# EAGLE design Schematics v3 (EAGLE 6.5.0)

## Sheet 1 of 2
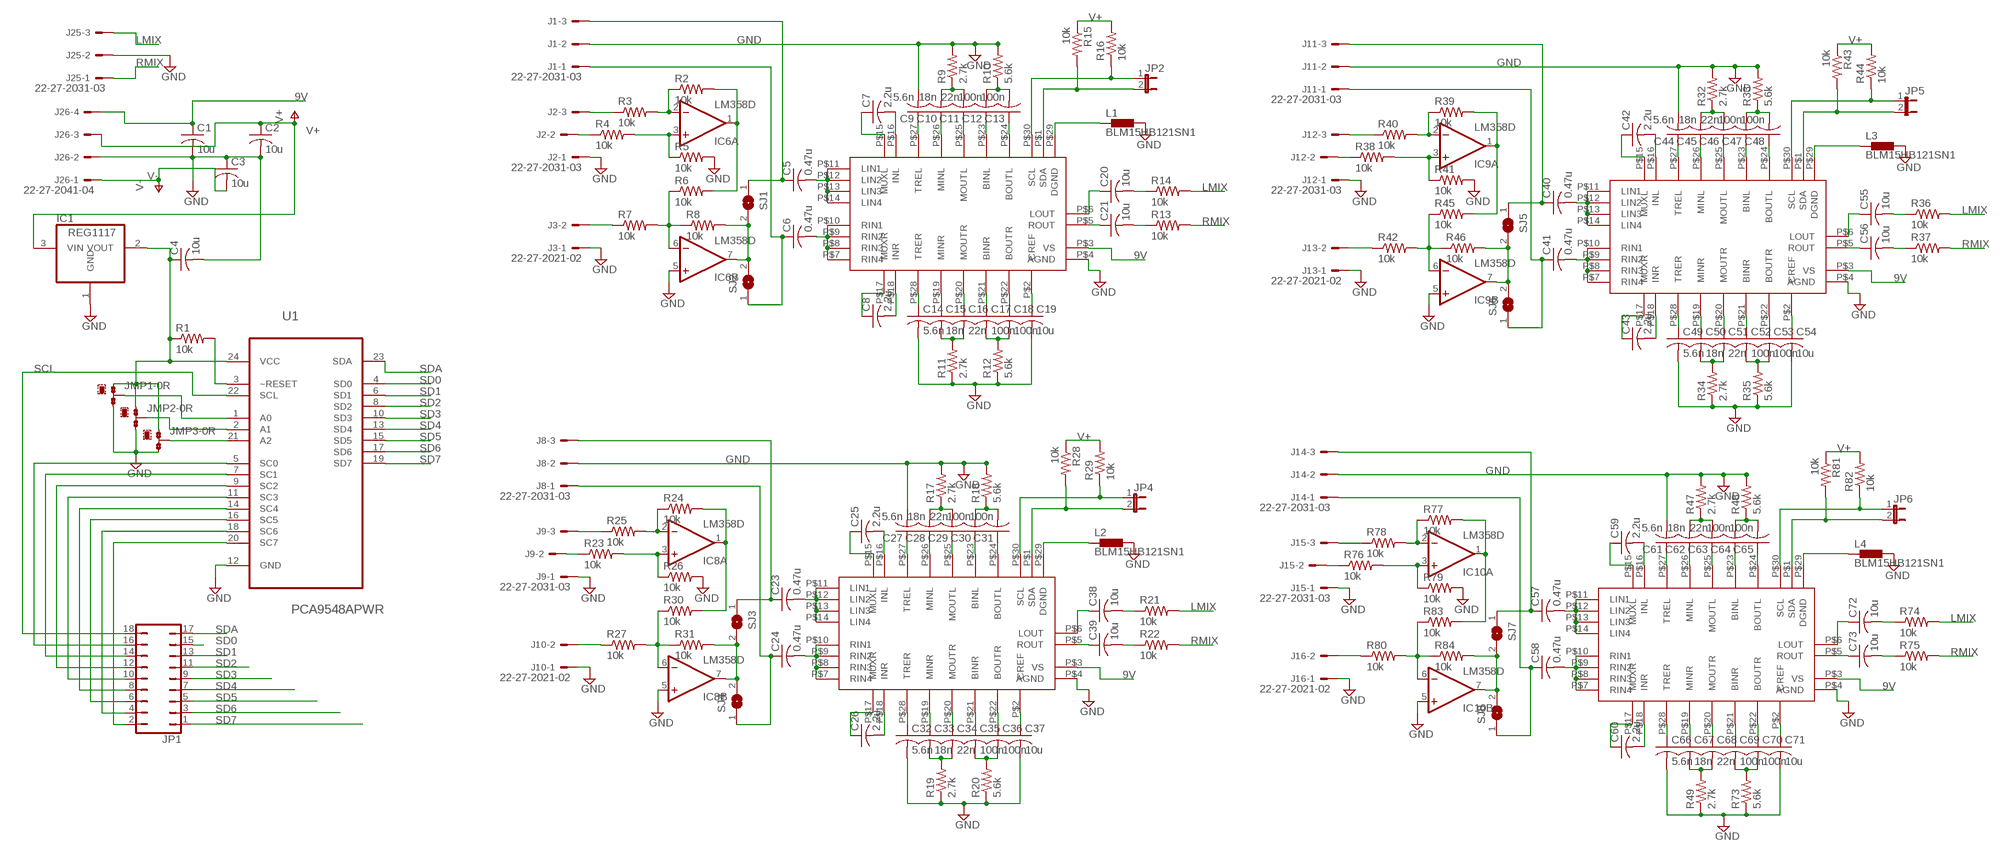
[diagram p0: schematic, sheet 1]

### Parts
C1  10u  C-USC1206  [C1206]
C2  10u  C-USC1206  [C1206]
C3  10u  C-USC1206  [C1206]
C4  10u  C-USC1206  [C1206]
C5  0.47u  C-USC1206  [C1206]
C6  0.47u  C-USC1206  [C1206]
C7  2.2u  C-USC1206  [C1206]
C8  2.2u  C-USC1206  [C1206]
C9  5.6n  C-USC1206  [C1206]
C10  18n  C-USC1206  [C1206]
C11  22n  C-USC1206  [C1206]
C12  100n  C-USC1206  [C1206]
C13  100n  C-USC1206  [C1206]
C14  5.6n  C-USC1206  [C1206]
C15  18n  C-USC1206  [C1206]
C16  22n  C-USC1206  [C1206]
C17  100n  C-USC1206  [C1206]
C18  100n  C-USC1206  [C1206]
C19  10u  C-USC1206  [C1206]
C20  10u  C-USC1206  [C1206]
C21  10u  C-USC1206  [C1206]
C23  0.47u  C-USC1206  [C1206]
C24  0.47u  C-USC1206  [C1206]
C25  2.2u  C-USC1206  [C1206]
C26  2.2u  C-USC1206  [C1206]
C27  5.6n  C-USC1206  [C1206]
C28  18n  C-USC1206  [C1206]
C29  22n  C-USC1206  [C1206]
C30  100n  C-USC1206  [C1206]
C31  100n  C-USC1206  [C1206]
C32  5.6n  C-USC1206  [C1206]
C33  18n  C-USC1206  [C1206]
C34  22n  C-USC1206  [C1206]
C35  100n  C-USC1206  [C1206]
C36  100n  C-USC1206  [C1206]
C37  10u  C-USC1206  [C1206]
C38  10u  C-USC1206  [C1206]
C39  10u  C-USC1206  [C1206]
C40  0.47u  C-USC1206  [C1206]
C41  0.47u  C-USC1206  [C1206]
C42  2.2u  C-USC1206  [C1206]
C43  2.2u  C-USC1206  [C1206]
C44  5.6n  C-USC1206  [C1206]
C45  18n  C-USC1206  [C1206]
C46  22n  C-USC1206  [C1206]
C47  100n  C-USC1206  [C1206]
C48  100n  C-USC1206  [C1206]
C49  5.6n  C-USC1206  [C1206]
C50  18n  C-USC1206  [C1206]
C51  22n  C-USC1206  [C1206]
C52  100n  C-USC1206  [C1206]
C53  100n  C-USC1206  [C1206]
C54  10u  C-USC1206  [C1206]
C55  10u  C-USC1206  [C1206]
C56  10u  C-USC1206  [C1206]
C57  0.47u  C-USC1206  [C1206]
C58  0.47u  C-USC1206  [C1206]
C59  2.2u  C-USC1206  [C1206]
C60  2.2u  C-USC1206  [C1206]
C61  5.6n  C-USC1206  [C1206]
C62  18n  C-USC1206  [C1206]
C63  22n  C-USC1206  [C1206]
C64  100n  C-USC1206  [C1206]
C65  100n  C-USC1206  [C1206]
C66  5.6n  C-USC1206  [C1206]
C67  18n  C-USC1206  [C1206]
C68  22n  C-USC1206  [C1206]
C69  100n  C-USC1206  [C1206]
C70  100n  C-USC1206  [C1206]
C71  10u  C-USC1206  [C1206]
C72  10u  C-USC1206  [C1206]
C73  10u  C-USC1206  [C1206]
IC1  REG1117  [SOT223]
IC6  LM358D  [SO08]
IC8  LM358D  [SO08]
IC9  LM358D  [SO08]
IC10  LM358D  [SO08]
J1  22-27-2031-03  [6410-03]
J2  22-27-2031-03  [6410-03]
J3  22-27-2021-02  [6410-02]
J8  22-27-2031-03  [6410-03]
J9  22-27-2031-03  [6410-03]
J10  22-27-2021-02  [6410-02]
J11  22-27-2031-03  [6410-03]
J12  22-27-2031-03  [6410-03]
J13  22-27-2021-02  [6410-02]
J14  22-27-2031-03  [6410-03]
J15  22-27-2031-03  [6410-03]
J16  22-27-2021-02  [6410-02]
J25  22-27-2031-03  [6410-03]
J26  22-27-2041-04  [6410-04]
JMP1  0R-JUMPB  [B0R-JMP]
JMP2  0R-JUMPB  [B0R-JMP]
JMP3  0R-JUMPB  [B0R-JMP]
JP1  JP9Q  [JP9Q]
JP2  JP1E  [JP1]
JP4  JP1E  [JP1]
JP5  JP1E  [JP1]
JP6  JP1E  [JP1]
L1  BLM15HB121SN1  [0402]
L2  BLM15HB121SN1  [0402]
L3  BLM15HB121SN1  [0402]
L4  BLM15HB121SN1  [0402]
R1  10k  R-US_R1206  [R1206]
R2  10k  R-US_R1206  [R1206]
R3  10k  R-US_R1206  [R1206]
R4  10k  R-US_R1206  [R1206]
R5  10k  R-US_R1206  [R1206]
R6  10k  R-US_R1206  [R1206]
R7  10k  R-US_R1206  [R1206]
R8  10k  R-US_R1206  [R1206]
R9  2.7k  R-US_R1206  [R1206]
R10  5.6k  R-US_R1206  [R1206]
R11  2.7k  R-US_R1206  [R1206]
R12  5.6k  R-US_R1206  [R1206]
R13  10k  R-US_R1206  [R1206]
R14  10k  R-US_R1206  [R1206]
R15  10k  R-US_R1206  [R1206]
R16  10k  R-US_R1206  [R1206]
R17  2.7k  R-US_R1206  [R1206]
R18  5.6k  R-US_R1206  [R1206]
R19  2.7k  R-US_R1206  [R1206]
R20  5.6k  R-US_R1206  [R1206]
R21  10k  R-US_R1206  [R1206]
R22  10k  R-US_R1206  [R1206]
R23  10k  R-US_R1206  [R1206]
R24  10k  R-US_R1206  [R1206]
R25  10k  R-US_R1206  [R1206]
R26  10k  R-US_R1206  [R1206]
R27  10k  R-US_R1206  [R1206]
R28  10k  R-US_R1206  [R1206]
R29  10k  R-US_R1206  [R1206]
R30  10k  R-US_R1206  [R1206]
R31  10k  R-US_R1206  [R1206]
R32  2.7k  R-US_R1206  [R1206]
R33  5.6k  R-US_R1206  [R1206]
R34  2.7k  R-US_R1206  [R1206]
R35  5.6k  R-US_R1206  [R1206]
R36  10k  R-US_R1206  [R1206]
R37  10k  R-US_R1206  [R1206]
R38  10k  R-US_R1206  [R1206]
R39  10k  R-US_R1206  [R1206]
R40  10k  R-US_R1206  [R1206]
R41  10k  R-US_R1206  [R1206]
R42  10k  R-US_R1206  [R1206]
R43  10k  R-US_R1206  [R1206]
R44  10k  R-US_R1206  [R1206]
R45  10k  R-US_R1206  [R1206]
R46  10k  R-US_R1206  [R1206]
R47  2.7k  R-US_R1206  [R1206]
R48  5.6k  R-US_R1206  [R1206]
R49  2.7k  R-US_R1206  [R1206]
R73  5.6k  R-US_R1206  [R1206]
R74  10k  R-US_R1206  [R1206]
R75  10k  R-US_R1206  [R1206]
R76  10k  R-US_R1206  [R1206]
R77  10k  R-US_R1206  [R1206]
R78  10k  R-US_R1206  [R1206]
R79  10k  R-US_R1206  [R1206]
R80  10k  R-US_R1206  [R1206]
R81  10k  R-US_R1206  [R1206]
R82  10k  R-US_R1206  [R1206]
R83  10k  R-US_R1206  [R1206]
R84  10k  R-US_R1206  [R1206]
SJ1  SJ  [SJ]
SJ2  SJ  [SJ]
SJ3  SJ  [SJ]
SJ4  SJ  [SJ]
SJ5  SJ  [SJ]
SJ6  SJ  [SJ]
SJ7  SJ  [SJ]
SJ8  SJ  [SJ]
U1  PCA9548APWR  [SOP65P640X120-24N]
U$1  TDA7439  [SDIP30]
U$2  TDA7439  [SDIP30]
U$3  TDA7439  [SDIP30]
U$4  TDA7439  [SDIP30]

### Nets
3.3V: C4.1 IC1.2(VOUT) JMP1.1 JMP2.1 JMP3.1 R1.1 U1.24(VCC)
9V: C1.1 J26.4 U$1.P$3(VS) U$2.P$3(VS) U$3.P$3(VS) U$4.P$3(VS) ; also sheet 2
A0: JMP1.2 U1.1(A0)
A1: JMP2.2 U1.2(A1)
A2: JMP3.2 U1.21(A2)
GND: C1.2 C2.2 C3.1 C4.2 C9.2 C14.2 C19.2 C27.2 C32.2 C37.2 C44.2 C49.2 C54.2 C61.2 C66.2 C71.2 IC1.1(GND) IC6.5(B:+IN) IC8.5(B:+IN) IC9.5(B:+IN) IC10.5(B:+IN) J1.2 J2.1 J3.1 J8.2 J9.1 J10.1 J11.2 J12.1 J13.1 J14.2 J15.1 J16.1 J25.2 J26.2 JMP1.3 JMP2.3 JMP3.3 L1.2 L2.2 L3.2 L4.2 R5.2 R9.2 R10.2 R11.1 R12.1 R17.2 R18.2 R19.1 R20.1 R26.2 R32.2 R33.2 R34.1 R35.1 R41.2 R47.2 R48.2 R49.1 R73.1 R79.2 U1.12(GND) U$1.P$4(AGND) U$2.P$4(AGND) U$3.P$4(AGND) U$4.P$4(AGND) ; also sheet 2
LMIX: J25.3 R14.2 R21.2 R36.2 R74.2 ; also sheet 2
N$1: J2.2 R4.1
N$2: J2.3 R3.1
N$3: IC6.2(A:-IN) R2.1 R3.2
N$4: IC6.3(A:+IN) R4.2 R5.1
N$5: IC6.1(A:OUT) R2.2 R6.2
N$6: IC6.6(B:-IN) R6.1 R7.2 R8.1
N$7: J3.2 R7.1
N$8: IC6.7(B:OUT) R8.2 SJ1.2 SJ2.2
N$9: C5.1 J1.3 SJ1.1
N$10: C6.1 J1.1 SJ2.1
N$11: C5.2 U$1.P$11(LIN1) U$1.P$12(LIN2) U$1.P$13(LIN3) U$1.P$14(LIN4)
N$12: C6.2 U$1.P$7(RIN4) U$1.P$8(RIN3) U$1.P$9(RIN2) U$1.P$10(RIN1)
N$13: C7.1 U$1.P$15(MUXL)
N$14: C7.2 U$1.P$16(INL)
N$15: C9.1 U$1.P$27(TREL)
N$16: C10.1 U$1.P$26(MINL)
N$17: C11.1 U$1.P$25(MOUTL)
N$18: C12.1 U$1.P$23(BINL)
N$19: C13.1 U$1.P$24(BOUTL)
N$20: C10.2 C11.2 R9.1
N$21: C12.2 C13.2 R10.1
N$22: C8.1 U$1.P$17(MUXR)
N$23: C8.2 U$1.P$18(INR)
N$24: C14.1 U$1.P$28(TRER)
N$25: C15.1 U$1.P$19(MINR)
N$26: C16.1 U$1.P$20(MOUTR)
N$27: C17.1 U$1.P$21(BINR)
N$28: C18.1 U$1.P$22(BOUTR)
N$29: C19.1 U$1.P$2(CREF)
N$30: C15.2 C16.2 R11.2
N$31: C17.2 C18.2 R12.2
N$32: JP2.1 R16.1 U$1.P$30(SCL)
N$33: JP2.2 R15.2 U$1.P$1(SDA)
N$34: L1.1 U$1.P$29(DGND)
N$35: C20.1 U$1.P$6(LOUT)
N$36: C21.1 U$1.P$5(ROUT)
N$37: C20.2 R14.1
N$38: C21.2 R13.1
N$46: J9.2 R23.1
N$47: J9.3 R25.1
N$48: IC8.2(A:-IN) R24.1 R25.2
N$49: IC8.3(A:+IN) R23.2 R26.1
N$50: IC8.1(A:OUT) R24.2 R30.2
N$51: IC8.6(B:-IN) R27.2 R30.1 R31.1
N$52: J10.2 R27.1
N$53: IC8.7(B:OUT) R31.2 SJ3.2 SJ4.2
N$54: C23.1 J8.3 SJ3.1
N$55: C24.1 J8.1 SJ4.1
N$56: C23.2 U$2.P$11(LIN1) U$2.P$12(LIN2) U$2.P$13(LIN3) U$2.P$14(LIN4)
N$57: C24.2 U$2.P$7(RIN4) U$2.P$8(RIN3) U$2.P$9(RIN2) U$2.P$10(RIN1)
N$58: C25.1 U$2.P$15(MUXL)
N$59: C25.2 U$2.P$16(INL)
N$60: C27.1 U$2.P$27(TREL)
N$61: C28.1 U$2.P$26(MINL)
N$62: C29.1 U$2.P$25(MOUTL)
N$63: C30.1 U$2.P$23(BINL)
N$64: C31.1 U$2.P$24(BOUTL)
N$65: C28.2 C29.2 R17.1
N$66: C30.2 C31.2 R18.1
N$67: C26.1 U$2.P$17(MUXR)
N$68: C26.2 U$2.P$18(INR)
N$69: C32.1 U$2.P$28(TRER)
N$70: C33.1 U$2.P$19(MINR)
N$71: C34.1 U$2.P$20(MOUTR)
N$72: C35.1 U$2.P$21(BINR)
N$73: C36.1 U$2.P$22(BOUTR)
N$74: C37.1 U$2.P$2(CREF)
N$75: C33.2 C34.2 R19.2
N$76: C35.2 C36.2 R20.2
N$77: JP4.1 R29.1 U$2.P$30(SCL)
N$78: JP4.2 R28.2 U$2.P$1(SDA)
N$79: L2.1 U$2.P$29(DGND)
N$80: C38.1 U$2.P$6(LOUT)
N$81: C39.1 U$2.P$5(ROUT)
N$82: C38.2 R21.1
N$83: C39.2 R22.1
N$84: J12.2 R38.1
N$85: J12.3 R40.1
N$86: IC9.2(A:-IN) R39.1 R40.2
N$87: IC9.3(A:+IN) R38.2 R41.1
N$88: IC9.1(A:OUT) R39.2 R45.2
N$89: IC9.6(B:-IN) R42.2 R45.1 R46.1
N$90: J13.2 R42.1
N$91: IC9.7(B:OUT) R46.2 SJ5.2 SJ6.2
N$92: C40.1 J11.3 SJ5.1
N$93: C41.1 J11.1 SJ6.1
N$94: C40.2 U$3.P$11(LIN1) U$3.P$12(LIN2) U$3.P$13(LIN3) U$3.P$14(LIN4)
N$95: C41.2 U$3.P$7(RIN4) U$3.P$8(RIN3) U$3.P$9(RIN2) U$3.P$10(RIN1)
N$96: C42.1 U$3.P$15(MUXL)
N$97: C42.2 U$3.P$16(INL)
N$98: C44.1 U$3.P$27(TREL)
N$99: C45.1 U$3.P$26(MINL)
N$100: C46.1 U$3.P$25(MOUTL)
N$101: C47.1 U$3.P$23(BINL)
N$102: C48.1 U$3.P$24(BOUTL)
N$103: C45.2 C46.2 R32.1
N$104: C47.2 C48.2 R33.1
N$105: C43.1 U$3.P$17(MUXR)
N$106: C43.2 U$3.P$18(INR)
N$107: C49.1 U$3.P$28(TRER)
N$108: C50.1 U$3.P$19(MINR)
N$109: C51.1 U$3.P$20(MOUTR)
N$110: C52.1 U$3.P$21(BINR)
N$111: C53.1 U$3.P$22(BOUTR)
N$112: C54.1 U$3.P$2(CREF)
N$113: C50.2 C51.2 R34.2
N$114: C52.2 C53.2 R35.2
N$115: JP5.1 R44.1 U$3.P$30(SCL)
N$116: JP5.2 R43.2 U$3.P$1(SDA)
N$117: L3.1 U$3.P$29(DGND)
N$118: C55.1 U$3.P$6(LOUT)
N$119: C56.1 U$3.P$5(ROUT)
N$120: C55.2 R36.1
N$121: C56.2 R37.1
N$122: J15.2 R76.1
N$123: J15.3 R78.1
N$124: IC10.2(A:-IN) R77.1 R78.2
N$125: IC10.3(A:+IN) R76.2 R79.1
N$126: IC10.1(A:OUT) R77.2 R83.2
N$127: IC10.6(B:-IN) R80.2 R83.1 R84.1
N$128: J16.2 R80.1
N$129: IC10.7(B:OUT) R84.2 SJ7.2 SJ8.2
N$130: C57.1 J14.3 SJ7.1
N$131: C58.1 J14.1 SJ8.1
N$132: C57.2 U$4.P$11(LIN1) U$4.P$12(LIN2) U$4.P$13(LIN3) U$4.P$14(LIN4)
N$133: C58.2 U$4.P$7(RIN4) U$4.P$8(RIN3) U$4.P$9(RIN2) U$4.P$10(RIN1)
N$134: C59.1 U$4.P$15(MUXL)
N$135: C59.2 U$4.P$16(INL)
N$136: C61.1 U$4.P$27(TREL)
N$137: C62.1 U$4.P$26(MINL)
N$138: C63.1 U$4.P$25(MOUTL)
N$139: C64.1 U$4.P$23(BINL)
N$140: C65.1 U$4.P$24(BOUTL)
N$141: C62.2 C63.2 R47.1
N$142: C64.2 C65.2 R48.1
N$143: C60.1 U$4.P$17(MUXR)
N$144: C60.2 U$4.P$18(INR)
N$145: C66.1 U$4.P$28(TRER)
N$146: C67.1 U$4.P$19(MINR)
N$147: C68.1 U$4.P$20(MOUTR)
N$148: C69.1 U$4.P$21(BINR)
N$149: C70.1 U$4.P$22(BOUTR)
N$150: C71.1 U$4.P$2(CREF)
N$151: C67.2 C68.2 R49.2
N$152: C69.2 C70.2 R73.2
N$153: JP6.1 R82.1 U$4.P$30(SCL)
N$154: JP6.2 R81.2 U$4.P$1(SDA)
N$155: L4.1 U$4.P$29(DGND)
N$156: C72.1 U$4.P$6(LOUT)
N$157: C73.1 U$4.P$5(ROUT)
N$158: C72.2 R74.1
N$159: C73.2 R75.1
N$250: JP1.2 U1.20(SC7)
N$251: JP1.4 U1.18(SC6)
N$252: JP1.6 U1.16(SC5)
N$253: JP1.8 U1.14(SC4)
N$254: JP1.10 U1.11(SC3)
N$255: JP1.12 U1.9(SC2)
N$256: JP1.14 U1.7(SC1)
N$259: JP1.16 U1.5(SC0)
RMIX: J25.1 R13.2 R22.2 R37.2 R75.2 ; also sheet 2
RST: R1.2 U1.3(~RESET)
SCL: JP1.18 U1.22(SCL)
SD0: JP1.15 U1.4(SD0) ; also sheet 2
SD1: JP1.13 U1.6(SD1) ; also sheet 2
SD2: JP1.11 U1.8(SD2)
SD3: JP1.9 U1.10(SD3)
SD4: JP1.7 U1.13(SD4)
SD5: JP1.5 U1.15(SD5)
SD6: JP1.3 U1.17(SD6)
SD7: JP1.1 U1.19(SD7)
SDA: JP1.17 U1.23(SDA)
V+: C2.1 IC1.3(VIN) J26.3 R15.1 R16.2 R28.1 R29.2 R43.1 R44.2 R81.1 R82.2
V-: C3.2 J26.1 ; also sheet 2

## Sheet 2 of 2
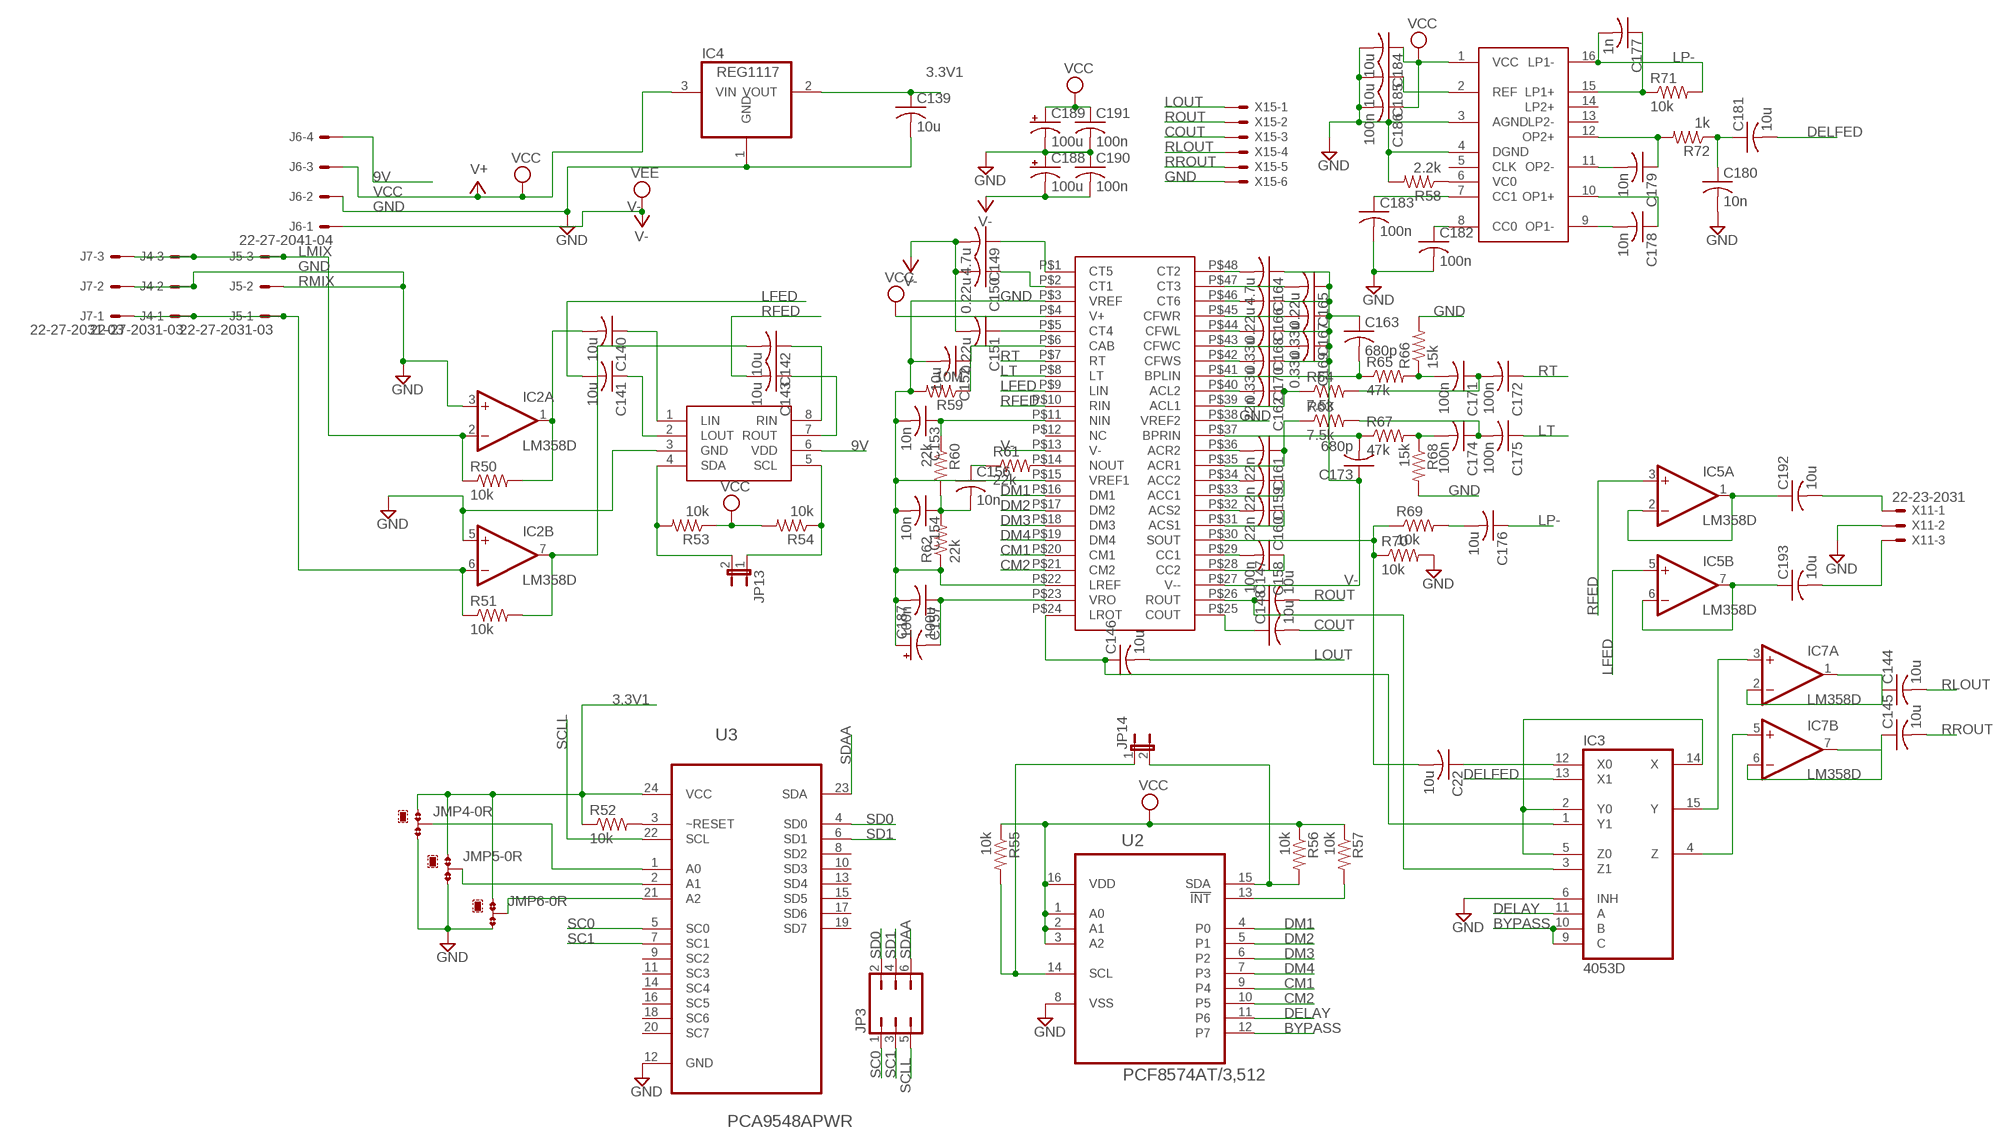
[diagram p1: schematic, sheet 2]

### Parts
C22  10u  C-USC1206  [C1206]
C139  10u  C-USC1206  [C1206]
C140  10u  C-USC1206  [C1206]
C141  10u  C-USC1206  [C1206]
C142  10u  C-USC1206  [C1206]
C143  10u  C-USC1206  [C1206]
C144  10u  C-USC1206  [C1206]
C145  10u  C-USC1206  [C1206]
C146  10u  C-USC1206  [C1206]
C147  10u  C-USC1206  [C1206]
C148  10u  C-USC1206  [C1206]
C149  4.7u  C-USC1206  [C1206]
C150  0.22u  C-USC1206  [C1206]
C151  0.22u  C-USC1206  [C1206]
C152  10u  C-USC1206  [C1206]
C153  10n  C-USC1206  [C1206]
C154  10n  C-USC1206  [C1206]
C156  10n  C-USC1206  [C1206]
C157  100n  C-USC1206  [C1206]
C158  100n  C-USC1206  [C1206]
C159  22n  C-USC1206  [C1206]
C160  22n  C-USC1206  [C1206]
C161  22n  C-USC1206  [C1206]
C162  22n  C-USC1206  [C1206]
C163  680p  C-USC1206  [C1206]
C164  4.7u  C-USC1206  [C1206]
C165  0.22u  C-USC1206  [C1206]
C166  0.22u  C-USC1206  [C1206]
C167  0.33u  C-USC1206  [C1206]
C168  0.33u  C-USC1206  [C1206]
C169  0.33u  C-USC1206  [C1206]
C170  0.33u  C-USC1206  [C1206]
C171  100n  C-USC1206  [C1206]
C172  100n  C-USC1206  [C1206]
C173  680p  C-USC1206  [C1206]
C174  100n  C-USC1206  [C1206]
C175  100n  C-USC1206  [C1206]
C176  10u  C-USC1206  [C1206]
C177  1n  C-USC1206  [C1206]
C178  10n  C-USC1206  [C1206]
C179  10n  C-USC1206  [C1206]
C180  10n  C-USC1206  [C1206]
C181  10u  C-USC1206  [C1206]
C182  100n  C-USC1206  [C1206]
C183  100n  C-USC1206  [C1206]
C184  10u  C-USC1206  [C1206]
C185  10u  C-USC1206  [C1206]
C186  100n  C-USC1206  [C1206]
C187  100u  CPOL-USE2-5  [E2-5]
C188  100u  CPOL-USE2-5  [E2-5]
C189  100u  CPOL-USE2-5  [E2-5]
C190  100n  C-USC1206  [C1206]
C191  100n  C-USC1206  [C1206]
C192  10u  C-USC1206  [C1206]
C193  10u  C-USC1206  [C1206]
IC2  LM358D  [SO08]
IC3  4053D  [SO16]
IC4  REG1117  [SOT223]
IC5  LM358D  [SO08]
IC7  LM358D  [SO08]
J4  22-27-2031-03  [6410-03]
J5  22-27-2031-03  [6410-03]
J6  22-27-2041-04  [6410-04]
J7  22-27-2031-03  [6410-03]
JMP4  0R-JUMPB  [B0R-JMP]
JMP5  0R-JUMPB  [B0R-JMP]
JMP6  0R-JUMPB  [B0R-JMP]
JP3  JP3Q  [JP3Q]
JP13  JP1E  [JP1]
JP14  JP1E  [JP1]
R50  10k  R-US_R1206  [R1206]
R51  10k  R-US_R1206  [R1206]
R52  10k  R-US_R1206  [R1206]
R53  10k  R-US_R1206  [R1206]
R54  10k  R-US_R1206  [R1206]
R55  10k  R-US_R1206  [R1206]
R56  10k  R-US_R1206  [R1206]
R57  10k  R-US_R1206  [R1206]
R58  2.2k  R-US_R1206  [R1206]
R59  10M  R-US_R1206  [R1206]
R60  22k  R-US_R1206  [R1206]
R61  22k  R-US_R1206  [R1206]
R62  22k  R-US_R1206  [R1206]
R63  7.5k  R-US_R1206  [R1206]
R64  7.5k  R-US_R1206  [R1206]
R65  47k  R-US_R1206  [R1206]
R66  15k  R-US_R1206  [R1206]
R67  47k  R-US_R1206  [R1206]
R68  15k  R-US_R1206  [R1206]
R69  10k  R-US_R1206  [R1206]
R70  10k  R-US_R1206  [R1206]
R71  10k  R-US_R1206  [R1206]
R72  1k  R-US_R1206  [R1206]
U2  PCF8574AT/3,512  [SOIC127P1032X265-16N]
U3  PCA9548APWR  [SOP65P640X120-24N]
U$9  SSM2126  [DIP48]
U$10  PT2257  [SO08]
U$11  PT2399  [DIL16]
X11  22-23-2031  [22-23-2031]
X15  22-23-2061  [22-23-2061]

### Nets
3.3V1: C139.1 IC4.2(VOUT) JMP4.1 JMP5.1 JMP6.1 R52.1 U3.24(VCC)
9V: J6.4 U$10.6(VDD) ; also sheet 1
BYPASS: IC3.9(C) IC3.10(B) U2.12(P7)
CM1: U2.9(P4) U$9.P$20(CM1)
CM2: U2.10(P5) U$9.P$21(CM2)
COUT: C148.2 X15.3
DELAY: IC3.11(A) U2.11(P6)
DELFED: C181.2 IC3.13(X1)
DM1: U2.4(P0) U$9.P$16(DM1)
DM2: U2.5(P1) U$9.P$17(DM2)
DM3: U2.6(P2) U$9.P$18(DM3)
DM4: U2.7(P3) U$9.P$19(DM4)
GND: C139.2 C152.2 C153.2 C154.2 C157.2 C180.2 C182.2 C183.2 C184.2 C185.2 C186.2 C187.+ C188.+ C189.- C190.1 C191.2 IC2.3(A:+IN) IC2.5(B:+IN) IC3.6(INH) IC4.1(GND) J4.2 J5.2 J6.2 J7.2 JMP4.3 JMP5.3 JMP6.3 R58.2 R59.2 R62.1 R66.2 R68.2 R70.2 U2.8(VSS) U3.12(GND) U$9.P$3(VREF) U$9.P$15(VREF1) U$9.P$22(LREF) U$9.P$38(VREF2) U$10.3(GND) U$11.3(AGND) U$11.4(DGND) X11.2 X15.6 ; also sheet 1
LFED: C141.2 IC5.5(B:+IN) U$9.P$9(LIN)
LMIX: IC2.2(A:-IN) J4.3 J5.3 J7.3 R50.1 ; also sheet 1
LOUT: C146.2 X15.1
LP-: C176.1 C177.2 R71.2 U$11.16(LP1-)
LT: C175.1 U$9.P$8(LT)
N$39: C22.1 IC3.12(X0)
N$40: C146.1 IC3.1(Y1) U$9.P$24(LROT)
N$41: C147.1 IC3.3(Z1) U$9.P$26(ROUT)
N$42: C144.1 IC7.1(A:OUT) IC7.2(A:-IN)
N$43: C145.1 IC7.6(B:-IN) IC7.7(B:OUT)
N$44: IC3.15(Y) IC7.3(A:+IN)
N$45: IC3.4(Z) IC7.5(B:+IN)
N$241: C140.2 IC2.1(A:OUT) R50.2
N$242: C192.1 IC5.1(A:OUT) IC5.2(A:-IN)
N$243: C193.1 IC5.6(B:-IN) IC5.7(B:OUT)
N$244: C142.2 IC2.7(B:OUT) R51.2
N$245: C140.1 U$10.1(LIN)
N$246: C142.1 U$10.8(RIN)
N$247: C141.1 U$10.2(LOUT)
N$248: C143.1 U$10.7(ROUT)
N$249: R52.2 U3.3(~RESET)
N$257: C192.2 X11.1
N$258: JMP5.2 U3.2(A1)
N$260: JMP6.2 U3.21(A2)
N$261: JMP4.2 U3.1(A0)
N$262: IC3.2(Y0) IC3.5(Z0) IC3.14(X)
N$263: R57.2 U2.13(!INT)
N$268: C148.1 U$9.P$25(COUT)
N$269: R58.1 U$11.6(VC0)
N$270: C149.1 U$9.P$1(CT5)
N$271: C150.1 U$9.P$2(CT1)
N$272: C151.1 U$9.P$5(CT4)
N$273: C152.1 R59.1 U$9.P$6(CAB)
N$274: R61.2 U$9.P$14(NOUT)
N$278: C153.1 R60.1 U$9.P$11(NIN)
N$279: C193.2 X11.3
N$281: C154.1 C156.2 R60.2 R62.2
N$282: C156.1 R61.1
N$283: C157.1 C187.- U$9.P$23(VRO)
N$284: C158.2 U$9.P$29(CC1)
N$285: C158.1 U$9.P$28(CC2)
N$286: C160.1 U$9.P$31(ACS1)
N$287: C160.2 U$9.P$32(ACS2)
N$289: C159.1 U$9.P$33(ACC1)
N$290: C159.2 U$9.P$34(ACC2)
N$291: C161.1 R63.1 U$9.P$35(ACR1)
N$292: C161.2 U$9.P$36(ACR2)
N$293: C162.2 U$9.P$40(ACL2)
N$294: C162.1 R64.1 U$9.P$39(ACL1)
N$295: C163.2 R65.1 U$9.P$41(BPLIN)
N$296: C166.2 U$9.P$46(CT6)
N$297: C170.2 U$9.P$42(CFWS)
N$298: C169.2 U$9.P$43(CFWC)
N$299: C168.2 U$9.P$44(CFWL)
N$300: C167.2 U$9.P$45(CFWR)
N$301: C165.2 U$9.P$47(CT3)
N$302: C164.2 U$9.P$48(CT2)
N$303: C171.2 R65.2 R66.1
N$304: C171.1 C172.2 R64.2
N$305: C173.2 R67.1 U$9.P$37(BPRIN)
N$306: C174.2 R67.2 R68.1
N$307: C174.1 C175.2 R63.2
N$308: C176.2 R69.2
N$309: C177.1 R71.1 U$11.15(LP1+)
N$310: C178.2 U$11.9(OP1-)
N$311: C179.2 U$11.11(OP2-)
N$312: C178.1 U$11.10(OP1+)
N$313: C179.1 R72.2 U$11.12(OP2+)
N$314: C180.1 C181.1 R72.1
N$315: C183.1 U$11.7(CC1)
N$316: C182.1 U$11.8(CC0)
N$317: C185.1 U$11.2(REF)
N$318: JP13.2 R53.2 U$10.4(SDA)
N$319: JP13.1 R54.1 U$10.5(SCL)
N$320: JP14.2 R56.2 U2.15(SDA)
N$321: JP14.1 R55.2 U2.14(SCL)
RFED: C143.2 IC5.3(A:+IN) U$9.P$10(RIN)
RLOUT: C144.2 X15.4
RMIX: IC2.6(B:-IN) J4.1 J5.1 J7.1 R51.1 ; also sheet 1
ROUT: C147.2 X15.2
RROUT: C145.2 X15.5
RT: C172.1 U$9.P$7(RT)
SC0: JP3.1 U3.5(SC0)
SC1: JP3.3 U3.7(SC1)
SCLL: JP3.5 U3.22(SCL)
SD0: JP3.2 U3.4(SD0) ; also sheet 1
SD1: JP3.4 U3.6(SD1) ; also sheet 1
SDAA: JP3.6 U3.23(SDA)
SFED: C22.2 R69.1 R70.1 U$9.P$30(SOUT)
V-: C149.2 C150.2 C151.2 C163.1 C164.1 C165.1 C166.1 C167.1 C168.1 C169.1 C170.1 C173.1 C188.- C190.2 J6.1 U$9.P$13(V-) U$9.P$27(V--) ; supply symbol labelled VEE ; also sheet 1
VCC: C184.1 C186.1 C189.+ C191.1 IC4.3(VIN) J6.3 R53.1 R54.2 R55.1 R56.1 R57.1 U2.1(A0) U2.2(A1) U2.3(A2) U2.16(VDD) U$9.P$4(V+) U$11.1(VCC) ; supply symbol labelled V+
Unconnected: U3.8(SD2) U3.9(SC2) U3.10(SD3) U3.11(SC3) U3.13(SD4) U3.14(SC4) U3.15(SD5) U3.16(SC5) U3.17(SD6) U3.18(SC6) U3.19(SD7) U3.20(SC7) U$9.P$12(NC) U$11.5(CLK) U$11.13(LP2-) U$11.14(LP2+)

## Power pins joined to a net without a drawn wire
GND: IC3.8(GND)
V+: IC6.8(P:V+) IC8.8(P:V+) IC9.8(P:V+) IC10.8(P:V+)
V-: IC2.4(P:V-) IC3.7(VEE) IC5.4(P:V-) IC6.4(P:V-) IC7.4(P:V-) IC8.4(P:V-) IC9.4(P:V-) IC10.4(P:V-)
VCC: IC2.8(P:V+) IC3.16(VCC) IC5.8(P:V+) IC7.8(P:V+)

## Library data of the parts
C1-C73 C139-C154 C156-C186 C190-C193 = adafruit:C-US: CAPACITOR, American symbol
C187-C189 = adafruit:CPOL-US: POLARIZED CAPACITOR, American symbol
IC1 IC4 = burr-brown:REG1117: 800mA and 1A Low Dropout (LDO) Positive Regulator 1.8V, 2.5V, 2.85V, 3.3V, 5V, and Adj; MPN: REG1117; OC_FARNELL: 1097566; OC_NEWARK: 14P6981
IC2 IC5-IC10 = linear:LM358: OP AMP also LM158; LM258; LM2904 Source: http://cache.national.com/ds/LM/LM158.pdf
IC3 = 40xx:4053: Triple 2-channel ANALOG MULTIPLEXER
J1 J2 J4 J5 J7-J9 J11 J12 J14 J15 J25 = con-molex:22-?-03: CONNECTOR wire to board 2.54 mm (.1 inch) pitch header; OC_FARNELL: unknown; OC_NEWARK: unknown
J3 J10 J13 J16 = con-molex:22-?-02: CONNECTOR; OC_FARNELL: unknown; OC_NEWARK: unknown
J6 J26 = con-molex:22-?-04: CONNECTOR wire to board 2.54 mm (.1 inch) pitch header; OC_FARNELL: unknown; OC_NEWARK: unknown
JMP1-JMP6 = jump-0r-smd:0R-JUMP: SMD 0R 0805 Jumper
JP1 = jumper:JP9Q: JUMPER
JP2 JP4-JP6 JP13 JP14 = jumper:JP1E: JUMPER
JP3 = jumper:JP3Q: JUMPER
L1-L4 = inductors:BLM15H: EMIFIL (R) Chip Ferrite Bead for GHz Noise
R1-R84 = adafruit:R-US_: RESISTOR, American symbol
SJ1-SJ8 = jumper:SJ: SMD solder JUMPER
U1 U3 = PCA9548A:PCA9548APWR: 8-CHANNEL I2C SWITCH WITH RESET; MPN: PCA9548APWR False; OC_FARNELL: 1607855; OC_NEWARK: 22M1602; PACKAGE: TSSOP-24; SUPPLIER: Texas Instruments
U2 = PCF8574A:PCF8574AT/3,512: IC, I/O EXPANDER, 8BIT, 16SOIC; MPN: PCF8574AT/3,512; OC_FARNELL: 2101302; OC_NEWARK: 70R6866; PACKAGE: SOIC-16; SUPPLIER: NXP
U$1-U$4 = adafruit:TDA7439
U$9 = adafruit:SSM2126
U$10 = adafruit:PT2257
U$11 = adafruit:PT2399
X11 = con-molex:22-23-2031: .100" (2.54mm) Center Header - 3 Pin; MF: MOLEX; MPN: 22-23-2031; OC_FARNELL: 1462950; OC_NEWARK: 30C0862
X15 = con-molex:22-23-2061: .100" (2.54mm) Center Header - 6 Pin; MF: MOLEX; MPN: 22-23-2061; OC_FARNELL: 1462922; OC_NEWARK: 27C1933

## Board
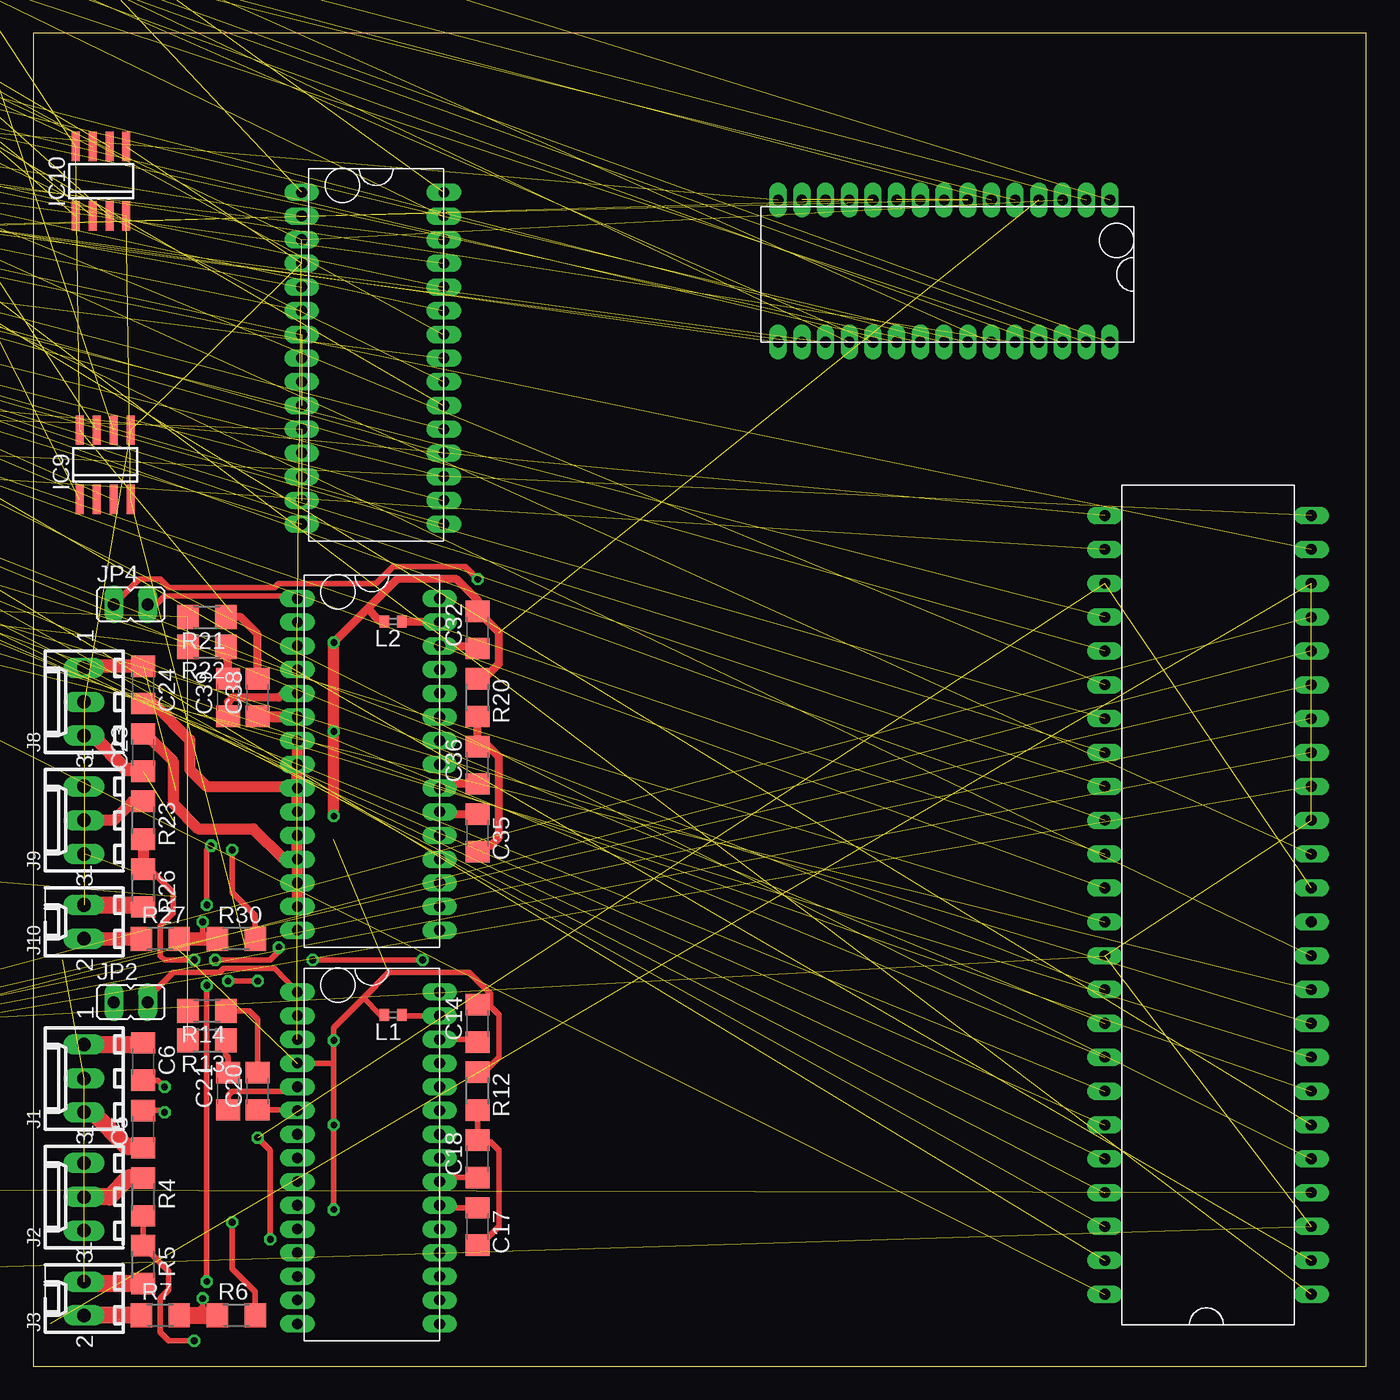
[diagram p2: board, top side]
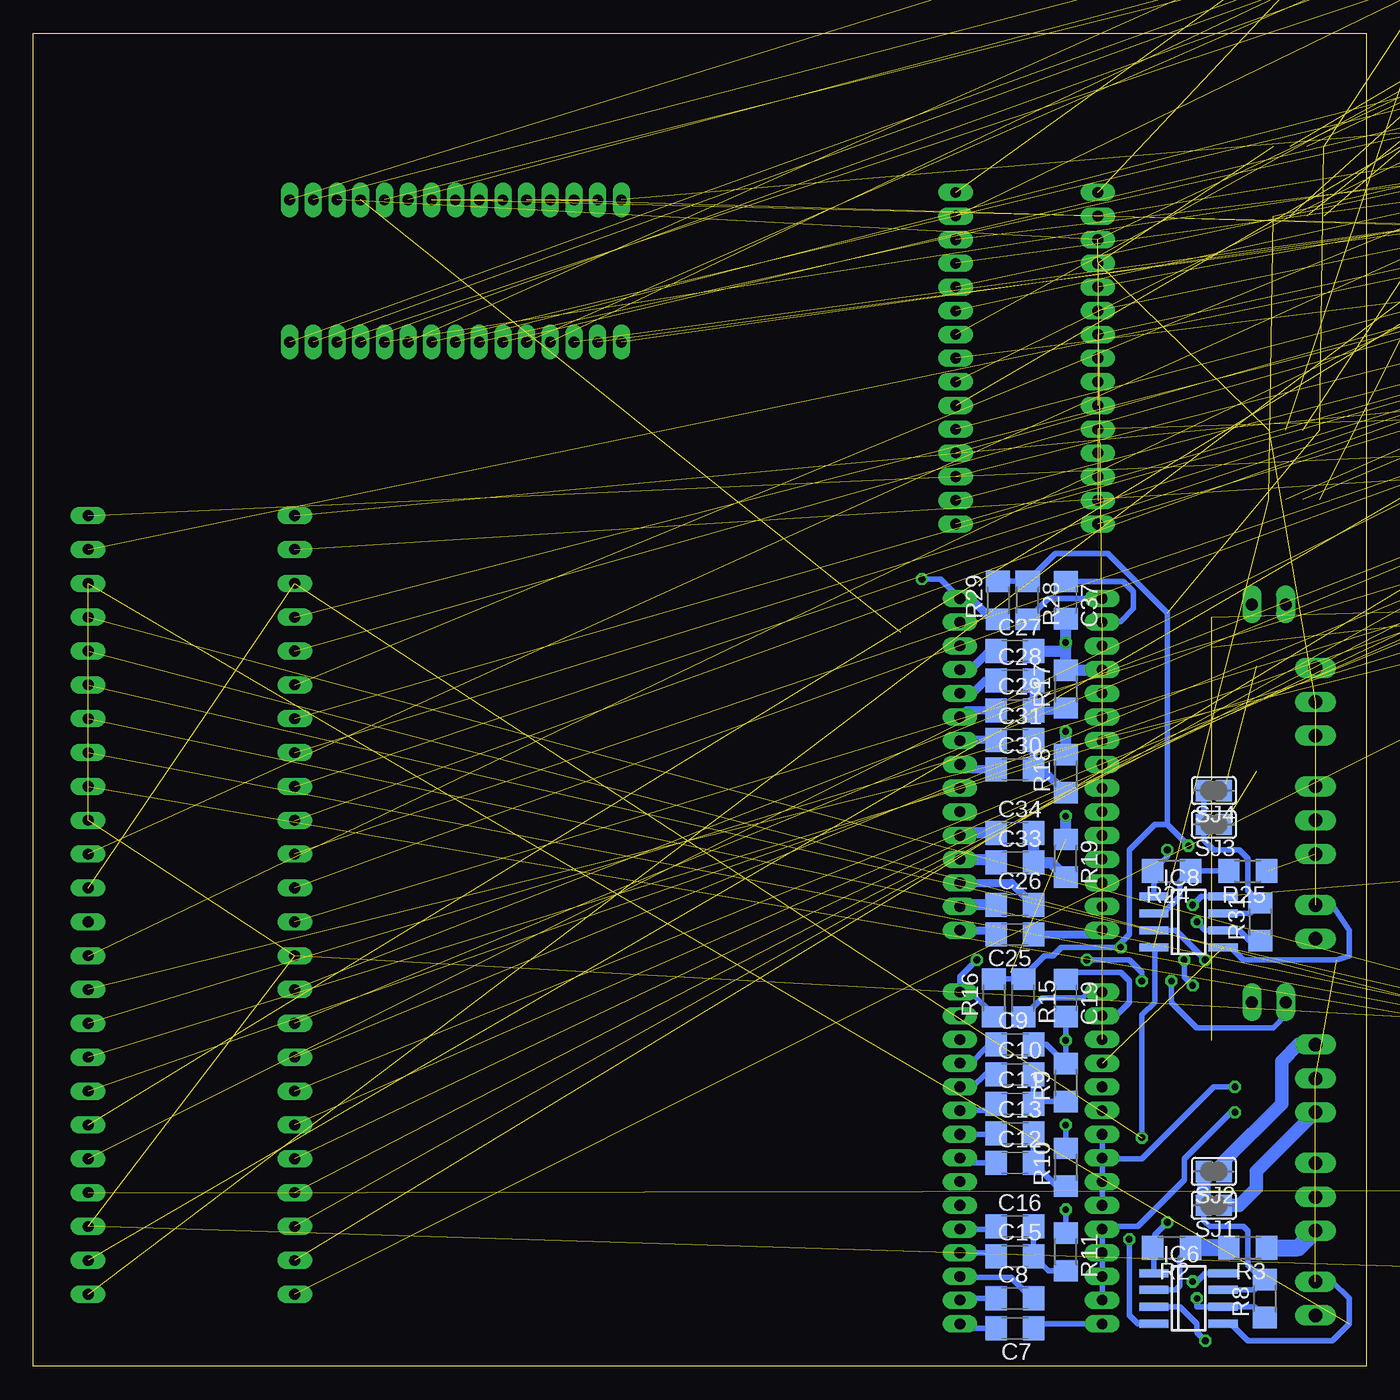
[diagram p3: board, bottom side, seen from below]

Size 100 x 100 mm. Coordinates in mm from the lower left corner, seen from the top.
Outline: 0,0 100,0 100,100 0,100 0,0
Copper layers (1*16): Top 0.035mm / dielectric 1.5mm / Bottom 0.035mm
Design rules "default": minimum track width 10mil, minimum drill 24mil, track to track 8mil, track to pad 8mil, pad to pad 8mil, via to via 8mil, smd to smd 8mil, copper to edge 40mil, drill to drill 8mil, minimum pad ring 10mil, minimum via ring 8mil, stop-mask expansion 4mil, vias tented up to drill 0mil, thermal gap 10mil

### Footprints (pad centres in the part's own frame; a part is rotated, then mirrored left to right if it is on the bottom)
C1206 = smd 1.6 x 1.8: 1 -1.4,0; 2 1.4,0
E2-5 = drill 0.813 pad 1.422: + -1.016,0 | drill 0.813 pad 1.422 octagon: - 1.016,0
SOT223 = smd 1.499 x 2.007: 1 -2.261,-3.15; 2 0.025,-3.15; 3 2.311,-3.15 | smd 3.81 x 2.007: 4 0,3.15
SO08 = smd 0.6 x 2.2: 1 -1.905,-2.6; 2 -0.635,-2.6; 3 0.635,-2.6; 4 1.905,-2.6; 5 1.905,2.6; 6 0.635,2.6; 7 -0.635,2.6; 8 -1.905,2.6
SO16 = smd 0.66 x 2.032: 1 -4.445,-3.073; 2 -3.175,-3.073; 3 -1.905,-3.073; 4 -0.635,-3.073; 5 0.635,-3.073; 6 1.905,-3.073; 7 3.175,-3.073; 8 4.445,-3.073; 9 4.445,3.073; 10 3.175,3.073; 11 1.905,3.073; 12 0.635,3.073; 13 -0.635,3.073; 14 -1.905,3.073; 15 -3.175,3.073; 16 -4.445,3.073
6410-03 = drill 1.016 long: 1 2.54,0; 2 0,0; 3 -2.54,0
6410-02 = drill 1.016 long: 1 1.27,0; 2 -1.27,0
6410-04 = drill 1.016 long: 1 3.81,0; 2 1.27,0; 3 -1.27,0; 4 -3.81,0
B0R-JMP = smd 1.5 x 1.3: 1 0,1.7; 2 0,0; 3 0,-1.7
JP9Q = drill 0.914 octagon: 1 -10.16,-1.27; 2 -10.16,1.27; 3 -7.62,-1.27; 4 -7.62,1.27; 5 -5.08,-1.27; 6 -5.08,1.27; 7 -2.54,-1.27; 8 -2.54,1.27; 9 0,-1.27; 10 0,1.27; 11 2.54,-1.27; 12 2.54,1.27; 13 5.08,-1.27; 14 5.08,1.27; 15 7.62,-1.27; 16 7.62,1.27; 17 10.16,-1.27; 18 10.16,1.27
JP1 = drill 0.914 long: 1 0,-1.27; 2 0,1.27
JP3Q = drill 0.914 octagon: 1 -2.54,-1.27; 2 -2.54,1.27; 3 0,-1.27; 4 0,1.27; 5 2.54,-1.27; 6 2.54,1.27
0402 = smd 0.7 x 0.9: 1 -0.65,0; 2 0.65,0
R1206 = smd 1.6 x 1.803: 1 -1.422,0; 2 1.422,0
SJ = smd 1.168 x 1.6: 1 -0.762,0; 2 0.762,0
SOP65P640X120-24N = smd 1.473 x 0.356: 1 -2.921,3.581; 2 -2.921,2.921; 3 -2.921,2.286; 4 -2.921,1.626; 5 -2.921,0.965; 6 -2.921,0.33; 7 -2.921,-0.33; 8 -2.921,-0.965; 9 -2.921,-1.626; 10 -2.921,-2.286; 11 -2.921,-2.921; 12 -2.921,-3.581; 13 2.921,-3.581; 14 2.921,-2.921; 15 2.921,-2.286; 16 2.921,-1.626; 17 2.921,-0.965; 18 2.921,-0.33; 19 2.921,0.33; 20 2.921,0.965; 21 2.921,1.626; 22 2.921,2.286; 23 2.921,2.921; 24 2.921,3.581
SOIC127P1032X265-16N = smd 2.286 x 0.559: 1 -4.521,4.445; 2 -4.521,3.175; 3 -4.521,1.905; 4 -4.521,0.635; 5 -4.521,-0.635; 6 -4.521,-1.905; 7 -4.521,-3.175; 8 -4.521,-4.445; 9 4.521,-4.445; 10 4.521,-3.175; 11 4.521,-1.905; 12 4.521,-0.635; 13 4.521,0.635; 14 4.521,1.905; 15 4.521,3.175; 16 4.521,4.445
SDIP30 = drill 0.8 long: P$1 1.778,-10.668; P$2 3.556,-10.668; P$3 5.334,-10.668; P$4 7.112,-10.668; P$5 8.89,-10.668; P$6 10.668,-10.668; P$7 12.446,-10.668; P$8 14.224,-10.668; P$9 16.002,-10.668; P$10 17.78,-10.668; P$11 19.558,-10.668; P$12 21.336,-10.668; P$13 23.114,-10.668; P$14 24.892,-10.668; P$15 26.67,-10.668; P$16 26.67,0; P$17 24.892,0; P$18 23.114,0; P$19 21.336,0; P$20 19.558,0; P$21 17.78,0; P$22 16.002,0; P$23 14.224,0; P$24 12.446,0; P$25 10.668,0; P$26 8.89,0; P$27 7.112,0; P$28 5.334,0; P$29 3.556,0; P$30 1.778,0
DIP48 = drill 0.8 long: P$1 -29.21,-8.89; P$2 -26.67,-8.89; P$3 -24.13,-8.89; P$4 -21.59,-8.89; P$5 -19.05,-8.89; P$6 -16.51,-8.89; P$7 -13.97,-8.89; P$8 -11.43,-8.89; P$9 -8.89,-8.89; P$10 -6.35,-8.89; P$11 -3.81,-8.89; P$12 -1.27,-8.89; P$13 1.27,-8.89; P$14 3.81,-8.89; P$15 6.35,-8.89; P$16 8.89,-8.89; P$17 11.43,-8.89; P$18 13.97,-8.89; P$19 16.51,-8.89; P$20 19.05,-8.89; P$21 21.59,-8.89; P$22 24.13,-8.89; P$23 26.67,-8.89; P$24 29.21,-8.89; P$25 29.21,6.604; P$26 26.67,6.604; P$27 24.13,6.604; P$28 21.59,6.604; P$29 19.05,6.604; P$30 16.51,6.604; P$31 13.97,6.604; P$32 11.43,6.604; P$33 8.89,6.604; P$34 6.35,6.604; P$35 3.81,6.604; P$36 1.27,6.604; P$37 -1.27,6.604; P$38 -3.81,6.604; P$39 -6.35,6.604; P$40 -8.89,6.604; P$41 -11.43,6.604; P$42 -13.97,6.604; P$43 -16.51,6.604; P$44 -19.05,6.604; P$45 -21.59,6.604; P$46 -24.13,6.604; P$47 -26.67,6.604; P$48 -29.21,6.604
SO08' = smd 0.66 x 2.032: 1 -1.905,-3.073; 2 -0.635,-3.073; 3 0.635,-3.073; 4 1.905,-3.073; 5 1.905,3.073; 6 0.635,3.073; 7 -0.635,3.073; 8 -1.905,3.073
DIL16 = drill 0.813 long: 1 -8.89,-3.81; 2 -6.35,-3.81; 3 -3.81,-3.81; 4 -1.27,-3.81; 5 1.27,-3.81; 6 3.81,-3.81; 7 6.35,-3.81; 8 8.89,-3.81; 9 8.89,3.81; 10 6.35,3.81; 11 3.81,3.81; 12 1.27,3.81; 13 -1.27,3.81; 14 -3.81,3.81; 15 -6.35,3.81; 16 -8.89,3.81
22-23-2031 = drill 1 long: 1 -2.54,0; 2 0,0; 3 2.54,0
22-23-2061 = drill 1 long: 1 -6.35,0; 2 -3.81,0; 3 -1.27,0; 4 1.27,0; 5 3.81,0; 6 6.35,0

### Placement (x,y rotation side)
C1  not placed on the board
C2  not placed on the board
C3  not placed on the board
C4  not placed on the board
C5  8.26,17.78 90 top
C6  8.26,22.86 270 top
C7  26.35,2.86 180 bottom
C8  26.35,5.08 0 bottom
C9  26.35,24.13 0 bottom
C10  26.35,21.91 0 bottom
C11  26.35,19.68 0 bottom
C12  26.35,15.24 0 bottom
C13  26.35,17.46 0 bottom
C14  33.34,25.72 90 top
C15  26.35,8.26 0 bottom
C16  26.35,10.48 0 bottom
C17  33.34,10.48 270 top
C18  33.34,15.56 90 top
C19  22.54,27.62 270 bottom
C20  16.83,20.64 90 top
C21  14.61,20.64 90 top
C22  not placed on the board
C23  8.26,46.04 90 top
C24  8.26,51.12 270 top
C25  26.35,32.38 180 bottom
C26  26.35,34.61 0 bottom
C27  26.35,53.66 0 bottom
C28  26.35,51.44 0 bottom
C29  26.35,49.21 0 bottom
C30  26.35,44.77 0 bottom
C31  26.35,46.99 0 bottom
C32  33.34,55.24 90 top
C33  26.35,37.78 0 bottom
C34  26.35,40.01 0 bottom
C35  33.34,40.01 270 top
C36  33.34,45.09 90 top
C37  22.54,57.47 270 bottom
C38  16.83,50.16 90 top
C39  14.61,50.16 90 top
C40  not placed on the board
C41  not placed on the board
C42  not placed on the board
C43  not placed on the board
C44  not placed on the board
C45  not placed on the board
C46  not placed on the board
C47  not placed on the board
C48  not placed on the board
C49  not placed on the board
C50  not placed on the board
C51  not placed on the board
C52  not placed on the board
C53  not placed on the board
C54  not placed on the board
C55  not placed on the board
C56  not placed on the board
C57  not placed on the board
C58  not placed on the board
C59  not placed on the board
C60  not placed on the board
C61  not placed on the board
C62  not placed on the board
C63  not placed on the board
C64  not placed on the board
C65  not placed on the board
C66  not placed on the board
C67  not placed on the board
C68  not placed on the board
C69  not placed on the board
C70  not placed on the board
C71  not placed on the board
C72  not placed on the board
C73  not placed on the board
C139  not placed on the board
C140  not placed on the board
C141  not placed on the board
C142  not placed on the board
C143  not placed on the board
C144  not placed on the board
C145  not placed on the board
C146  not placed on the board
C147  not placed on the board
C148  not placed on the board
C149  not placed on the board
C150  not placed on the board
C151  not placed on the board
C152  not placed on the board
C153  not placed on the board
C154  not placed on the board
C156  not placed on the board
C157  not placed on the board
C158  not placed on the board
C159  not placed on the board
C160  not placed on the board
C161  not placed on the board
C162  not placed on the board
C163  not placed on the board
C164  not placed on the board
C165  not placed on the board
C166  not placed on the board
C167  not placed on the board
C168  not placed on the board
C169  not placed on the board
C170  not placed on the board
C171  not placed on the board
C172  not placed on the board
C173  not placed on the board
C174  not placed on the board
C175  not placed on the board
C176  not placed on the board
C177  not placed on the board
C178  not placed on the board
C179  not placed on the board
C180  not placed on the board
C181  not placed on the board
C182  not placed on the board
C183  not placed on the board
C184  not placed on the board
C185  not placed on the board
C186  not placed on the board
C187  not placed on the board
C188  not placed on the board
C189  not placed on the board
C190  not placed on the board
C191  not placed on the board
C192  not placed on the board
C193  not placed on the board
IC1  not placed on the board
IC2  not placed on the board
IC3  not placed on the board
IC4  not placed on the board
IC5  not placed on the board
IC6  13.34,5.08 270 bottom
IC7  not placed on the board
IC8  13.34,33.34 270 bottom
IC9  5.4,67.63 0 top
IC10  5.08,88.9 0 top
J1  3.81,21.59 90 top
J2  3.81,12.7 90 top
J3  3.81,5.08 90 top
J4  not placed on the board
J5  not placed on the board
J6  not placed on the board
J7  not placed on the board
J8  3.81,49.85 90 top
J9  3.81,40.96 90 top
J10  3.81,33.34 90 top
J11  not placed on the board
J12  not placed on the board
J13  not placed on the board
J14  not placed on the board
J15  not placed on the board
J16  not placed on the board
J25  not placed on the board
J26  not placed on the board
JMP1  not placed on the board
JMP2  not placed on the board
JMP3  not placed on the board
JMP4  not placed on the board
JMP5  not placed on the board
JMP6  not placed on the board
JP1  not placed on the board
JP2  7.3,27.3 270 top
JP3  not placed on the board
JP4  7.3,57.15 270 top
JP5  not placed on the board
JP6  not placed on the board
JP13  not placed on the board
JP14  not placed on the board
L1  26.99,26.35 180 top
L2  26.99,55.88 180 top
L3  not placed on the board
L4  not placed on the board
R1  not placed on the board
R2  14.61,8.89 180 bottom
R3  8.89,8.89 180 bottom
R4  8.26,12.7 270 top
R5  8.26,7.62 270 top
R6  15.24,3.81 0 top
R7  9.53,3.81 0 top
R8  7.62,5.08 90 bottom
R9  22.54,21.27 90 bottom
R10  22.54,14.92 90 bottom
R11  22.54,8.57 270 bottom
R12  33.34,20.64 270 top
R13  13.02,24.45 180 top
R14  13.02,26.67 180 top
R15  25.72,27.62 270 bottom
R16  27.94,27.62 90 bottom
R17  22.54,50.8 90 bottom
R18  22.54,44.45 90 bottom
R19  22.54,38.1 270 bottom
R20  33.34,50.16 270 top
R21  13.02,56.2 180 top
R22  13.02,53.98 180 top
R23  8.26,40.96 270 top
R24  14.61,37.15 180 bottom
R25  8.89,37.15 180 bottom
R26  8.26,35.88 270 top
R27  9.53,32.07 0 top
R28  25.4,57.47 270 bottom
R29  27.62,57.47 90 bottom
R30  15.24,32.07 0 top
R31  7.94,33.34 90 bottom
R32  not placed on the board
R33  not placed on the board
R34  not placed on the board
R35  not placed on the board
R36  not placed on the board
R37  not placed on the board
R38  not placed on the board
R39  not placed on the board
R40  not placed on the board
R41  not placed on the board
R42  not placed on the board
R43  not placed on the board
R44  not placed on the board
R45  not placed on the board
R46  not placed on the board
R47  not placed on the board
R48  not placed on the board
R49  not placed on the board
R50  not placed on the board
R51  not placed on the board
R52  not placed on the board
R53  not placed on the board
R54  not placed on the board
R55  not placed on the board
R56  not placed on the board
R57  not placed on the board
R58  not placed on the board
R59  not placed on the board
R60  not placed on the board
R61  not placed on the board
R62  not placed on the board
R63  not placed on the board
R64  not placed on the board
R65  not placed on the board
R66  not placed on the board
R67  not placed on the board
R68  not placed on the board
R69  not placed on the board
R70  not placed on the board
R71  not placed on the board
R72  not placed on the board
R73  not placed on the board
R74  not placed on the board
R75  not placed on the board
R76  not placed on the board
R77  not placed on the board
R78  not placed on the board
R79  not placed on the board
R80  not placed on the board
R81  not placed on the board
R82  not placed on the board
R83  not placed on the board
R84  not placed on the board
SJ1  11.43,12.06 180 bottom
SJ2  11.43,14.61 180 bottom
SJ3  11.43,40.64 180 bottom
SJ4  11.43,43.18 180 bottom
SJ5  not placed on the board
SJ6  not placed on the board
SJ7  not placed on the board
SJ8  not placed on the board
U1  not placed on the board
U2  not placed on the board
U3  not placed on the board
U$1  30.48,29.84 270 top
U$2  30.48,59.37 270 top
U$3  30.8,89.85 270 top
U$4  82.55,76.83 180 top
U$9  87,34.61 90 top
U$10  PT2257  [SO08']  not placed on the board
U$11  not placed on the board
X11  not placed on the board
X15  not placed on the board

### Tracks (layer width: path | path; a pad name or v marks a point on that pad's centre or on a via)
3.3V  (6 unrouted)
3.3V1  (6 unrouted)
9V  (7 unrouted)
A0  (1 unrouted)
A1  (1 unrouted)
A2  (1 unrouted)
BYPASS  (2 unrouted)
CM1  (1 unrouted)
CM2  (1 unrouted)
COUT  (1 unrouted)
DELAY  (1 unrouted)
DELFED  (1 unrouted)
DM1  (1 unrouted)
DM2  (1 unrouted)
DM3  (1 unrouted)
DM4  (1 unrouted)
GND  (via drill 0.5)  (91 unrouted)
  Top 0.406: v22.54,11.75 v22.54,18.1 R9.2 | R9.2 v22.54,24.45 22.54,25.4 24.77,27.62 | U$1.P$4 22.5,22.73 R9.2 | R12.1 33.81,22.06 34.92,23.18 34.92,26.35 34.29,26.99 | 34.29,26.99 33.47,26.99 C14.2 | 34.29,26.99 34.29,27.94 32.7,29.53 26.67,29.53 24.77,27.62 | L1.2 26.04,26.35 24.77,27.62
  Top 0.61: R20.1 33.81,51.59 34.92,52.7 34.92,55.06 C32.2 33.34,57.47 31.75,59.05 27.3,59.05 25.08,56.83 | 25.08,56.83 v22.54,54.29 | L2.2 26.04,55.88 25.08,56.83
  Top 0.813: v22.54,54.29 v22.54,47.62 v22.54,41.27
  Top 1.27: R5.2 3.96,6.2 J3.1 | J10.1 8.1,34.61 R26.2
  Bottom 0.406: IC6.5 10.16,3.17 8.89,1.91 2.54,1.91 1.27,3.17 1.27,5.08 2.54,6.35 J3.1 | R11.1 v22.54,11.75 | v22.54,18.1 R10.2 | C9.2 23.98,24.13 R9.2 v22.54,24.45 C19.2 | IC8.5 10.16,31.43 9.21,30.48 2.22,30.48 1.27,30.8 1.27,32.7 2.54,34.61 J10.1
  Bottom 0.813: U$2.P$4 19.85,52.22 R17.2 22.54,53.66 | 22.54,53.66 v22.54,54.29 | v22.54,54.29 C37.2 | C27.2 22.86,53.66 | 22.86,53.66 22.54,53.66 | R18.2 v22.54,47.62 | v22.54,54.29 22.54,53.98 22.86,53.66 | R19.1 v22.54,41.27
LFED  (2 unrouted)
LMIX  (9 unrouted)
LOUT  (1 unrouted)
LP-  (3 unrouted)
LT  (1 unrouted)
N$1
  Top 1.27: R4.1 7.14,14.12 5.71,12.7 J2.2
N$2
  Bottom 1.27: R3.1 5.08,8.89 J2.3
N$3
  Bottom 0.406: 12.7,8.41 R2.1 13.97,8.1 13.97,6.03 14.29,5.71 IC6.2
  Bottom 1.27: R3.2 R2.1
N$4  (via drill 0.5)
  Top 0.406: v12.06,1.91 10.16,1.91 9.53,2.54 9.53,5.08 10.16,5.71 10.16,7.14 R5.1 R4.2
  Bottom 0.406: IC6.3 13.97,4.45 12.7,3.17 12.7,2.54 v12.06,1.91
N$5  (via drill 0.5)
  Top 0.406: R6.2 16.66,5.56 14.92,7.3 v14.92,10.79
  Bottom 0.406: 16.51,6.99 IC6.1 15.94,8.8 R2.2 15.88,9.04 15.88,9.84 v14.92,10.79
N$6  (via drill 0.5)
  Top 0.406: v12.7,5.08 12.7,4.45 12.06,3.81
  Top 1.27: R7.2 12.06,3.81 R6.1
  Bottom 0.406: v12.7,5.08 12.7,4.45 IC6.6 8.41,4.45 R8.1
N$7
  Top 1.27: R7.1 J3.2
N$8
  Bottom 0.406: IC6.7 8.41,5.71 R8.2 8.1,6.99 8.26,6.99 8.89,7.62 8.89,10.16 9.21,10.48 11.75,10.48 12.19,10.92 SJ1.2
  Bottom 1.016: SJ2.2 SJ1.2
N$9
  Top 1.27: J1.3 4.45,19.05 6.99,16.51 8.12,16.51 C5.1
  Bottom 1.016: SJ1.1 9.53,12.06 8.26,13.34 8.26,14.61 J1.3
N$10
  Top 1.27: J1.1 8.12,24.13 C6.1
  Bottom 1.016: SJ2.1 10.67,15.37 6.35,19.68 6.35,22.86 5.08,24.13 J1.1
N$11  (via drill 0.5)
  Top 0.406: C5.2 9.71,19.18 v9.84,19.05
  Bottom 0.406: v9.84,19.05 10.16,19.05 13.65,15.56 13.65,13.97 17.14,10.48 19.62,10.48 U$1.P$11 U$1.P$12 U$1.P$13 U$1.P$14
N$12  (via drill 0.5)
  Top 0.406: C6.2 9.34,21.46 v9.84,20.95
  Bottom 0.406: v9.84,20.95 11.43,20.95 16.83,15.56 19.75,15.56 U$1.P$8 | 19.75,17.46 U$1.P$7 U$1.P$8 | U$1.P$8 U$1.P$9 U$1.P$10
N$13
  Bottom 0.406: U$1.P$15 24.64,3.17 C7.1
N$14
  Bottom 0.406: C7.2 30.16,2.86 U$1.P$16
N$15
  Bottom 0.406: C9.1 28.26,24.13 29.84,22.54 30.29,22.54 U$1.P$27
N$16
  Bottom 0.406: U$1.P$26 29.53,20.95 28.57,21.91 C10.1
N$17
  Bottom 0.406: U$1.P$25 28.26,19.18 C11.1
N$18
  Bottom 0.406: C12.1 30.1,15.24 U$1.P$23
N$19
  Bottom 0.406: U$1.P$24 27.82,17.4 C13.1
N$20
  Bottom 0.406: C10.2 C11.2 24.79,19.85 R9.1
N$21
  Bottom 0.406: R10.1 23.21,13.5 C12.2 C13.2
N$22
  Bottom 0.406: C8.1 30.35,5.08 U$1.P$17
N$23
  Bottom 0.406: C8.2 25.08,5.08 26.67,6.67 30.42,6.67 U$1.P$18
N$24
  Top 0.406: U$1.P$28 33.14,24.51 C14.1
N$25
  Bottom 0.406: U$1.P$19 28.01,8.51 C15.1
N$26
  Bottom 0.406: U$1.P$20 27.94,10.29 C16.1
N$27
  Top 0.406: C17.1 30.67,11.88 U$1.P$21
N$28
  Top 0.406: C18.1 30.79,14.16 U$1.P$22
N$29
  Bottom 0.406: U$1.P$2 18.8,26.29 17.78,27.3 17.78,28.89 18.41,29.53 22.04,29.53 C19.1
N$30
  Bottom 0.406: C16.2 C15.2 23.85,7.15 R11.2
N$31
  Top 0.406: C17.2 33.52,9.08 34.92,10.48 34.92,16.19 34.29,16.83 33.47,16.83 C18.2 R12.2
N$32  (via drill 0.5)
  Top 0.406: v20.95,30.48 v29.21,30.48 | v16.83,28.89 v14.61,28.89
  Bottom 0.406: R16.1 27.94,26.35 29.53,27.94 30.35,27.94 U$1.P$30 30.48,29.21 v29.21,30.48 | JP2.1 6.03,26.35 6.99,25.4 12.7,25.4 14.61,27.3 v14.61,28.89 | v20.95,30.48 17.78,30.48 16.83,29.53 v16.83,28.89
N$33
  Top 0.406: JP2.2 8.57,27.62 10.48,29.53 13.97,29.53 14.29,29.84 18.1,29.84 19.94,27.94 U$1.P$1
  Bottom 0.406: U$1.P$1 20.83,28.07 21.27,27.62 24.3,27.62 R15.2
N$34
  Top 0.406: U$1.P$29 27.7,26.29 L1.1
N$35
  Top 0.406: C20.1 19.75,19.24 U$1.P$6
N$36
  Top 0.406: C21.1 14.61,20.32 14.92,20.64 19.49,20.64 U$1.P$5
N$37
  Top 0.406: C20.2 16.83,26.04 16.19,26.67 R14.1
N$38
  Top 0.406: C21.2 14.61,23.18 14.44,23.34 R13.1
N$39  (1 unrouted)
N$40  (2 unrouted)
N$41  (2 unrouted)
N$42  (2 unrouted)
N$43  (2 unrouted)
N$44  (1 unrouted)
N$45  (1 unrouted)
N$46
  Top 0.813: R23.1 7.46,42.38 6.03,40.96 J9.2
N$47  (1 unrouted)
N$48
  Bottom 0.406: IC8.2 15.24,33.97 13.97,35.24 13.97,36.36 R24.1 R25.2
N$49  (via drill 0.5)
  Top 0.406: R26.1 8.74,37.3 10.48,35.56 10.48,33.97 9.53,33.02 9.53,30.8 9.84,30.48 v12.06,30.48
  Top 0.813: R23.2 R26.1
  Bottom 0.406: IC8.3 14.29,32.7 v12.06,30.48
N$50  (via drill 0.5)
  Top 0.406: R30.2 16.66,33.82 14.92,35.56 v14.92,38.73
  Bottom 0.406: v14.92,38.73 14.92,38.25 R24.2 15.94,37.06 IC8.1
N$51  (via drill 0.5)
  Top 0.406: v12.7,33.34 12.7,32.07
  Top 1.016: R27.2 12.7,32.07 R30.1
  Bottom 0.406: R31.1 8.74,31.92 9.53,32.7 IC8.6 12.06,32.7 v12.7,33.34
N$52
  Top 1.016: J10.2 R27.1
N$53
  Bottom 0.406: IC8.7 8.72,33.97 R31.2 8.89,35.71 8.89,38.1 9.53,38.73 11.43,38.73 12.19,39.5 SJ4.2 SJ3.2
N$54  (1 unrouted)
  Top 1.016: J8.3 4.45,47.31 6.99,44.77 8.12,44.77 C23.1
N$55  (1 unrouted)
  Top 1.016: C24.1 3.94,52.52 J8.1
N$56
  Top 0.813: C23.2 8.44,47.44 10.48,45.4 10.48,42.23 12.38,40.32 16.51,40.32 18.73,38.1 19.75,38.1 U$2.P$12 | U$2.P$12 U$2.P$11 | U$2.P$14 U$2.P$13 U$2.P$12
N$57
  Top 0.813: C24.2 9.02,49.72 11.75,46.99 11.75,44.77 13.02,43.5 19.68,43.5 U$2.P$9 | U$2.P$7 U$2.P$8 U$2.P$9 | U$2.P$10 U$2.P$9
N$58
  Bottom 0.61: C25.1 20.13,32.38 U$2.P$15
N$59
  Bottom 0.61: U$2.P$16 28.07,32.7 C25.2
N$60
  Bottom 0.61: C27.1 28.26,53.66 29.84,52.07 30.29,52.07 U$2.P$27
N$61
  Bottom 0.61: C28.1 28.57,51.44 29.53,50.48 U$2.P$26
N$62
  Bottom 0.61: C29.1 29.97,49.21 U$2.P$25
N$63
  Bottom 0.61: C30.1 30.1,44.77 U$2.P$23
N$64
  Bottom 0.61: C31.1 30.42,46.99 U$2.P$24
N$65
  Bottom 0.61: C28.2 C29.2 22.71,49.21 R17.1
N$66
  Bottom 0.61: C31.2 C30.2 24.28,44.77 R18.1
N$67
  Bottom 0.813: C26.1 29.53,34.61 29.84,34.29 30.29,34.29 U$2.P$17
N$68
  Bottom 0.61: U$2.P$18 26.6,36.26 C26.2
N$69
  Top 0.61: U$2.P$28 33.14,54.04 C32.1
N$70
  Bottom 0.813: U$2.P$19 28.01,38.04 C33.1
N$71
  Bottom 0.813: C34.1 30.29,40.01 U$2.P$20
N$72
  Top 0.61: C35.1 30.67,41.41 U$2.P$21
N$73
  Top 0.61: C36.1 30.79,43.69 U$2.P$22
N$74
  Bottom 0.406: C37.1 18.23,58.87 17.46,58.1 17.46,56.83 18.41,55.88 19.75,55.88 U$2.P$2
N$75
  Bottom 0.813: R19.2 23.65,37.78 C33.2 C34.2
N$76
  Top 0.61: C35.2 33.34,38.73 33.02,39.05 34.29,39.05 34.92,39.69 34.92,45.72 33.97,46.67 33.52,46.67 C36.2 R20.2
N$77  (via drill 0.5)
  Top 0.406: JP4.1 6.03,57.47 6.35,57.78 6.67,57.78 7.94,59.05 9.53,59.05 10.16,58.42 18.1,58.42 18.41,58.74 25.72,58.74 26.99,60.01 32.38,60.01 v33.34,59.05
  Bottom 0.406: v33.34,59.05 31.94,59.05 U$2.P$30
  Bottom 0.61: R29.1 28.11,56.05 29.53,57.47 30.35,57.47 U$2.P$30
N$78
  Top 0.406: JP4.2 9.21,57.15 9.84,57.78 19.62,57.78 U$2.P$1
  Bottom 0.406: U$2.P$1 23.85,57.59 R28.2
N$79
  Top 0.61: U$2.P$29 27.7,55.82 L2.1
N$80
  Top 0.813: U$2.P$6 16.89,48.7 C38.1
N$81
  Top 0.61: U$2.P$5 18.73,50.48 18.41,50.16 14.92,50.16 14.61,49.85 C39.1
N$82
  Top 0.61: C38.2 16.83,54.93 15.56,56.2 R21.1
N$83
  Top 0.61: C39.2 14.61,52.7 R22.1
N$84  (1 unrouted)
N$85  (1 unrouted)
N$86  (2 unrouted)
N$87  (2 unrouted)
N$88  (2 unrouted)
N$89  (3 unrouted)
N$90  (1 unrouted)
N$91  (3 unrouted)
N$92  (2 unrouted)
N$93  (2 unrouted)
N$94  (4 unrouted)
N$95  (4 unrouted)
N$96  (1 unrouted)
N$97  (1 unrouted)
N$98  (1 unrouted)
N$99  (1 unrouted)
N$100  (1 unrouted)
N$101  (1 unrouted)
N$102  (1 unrouted)
N$103  (2 unrouted)
N$104  (2 unrouted)
N$105  (1 unrouted)
N$106  (1 unrouted)
N$107  (1 unrouted)
N$108  (1 unrouted)
N$109  (1 unrouted)
N$110  (1 unrouted)
N$111  (1 unrouted)
N$112  (1 unrouted)
N$113  (2 unrouted)
N$114  (2 unrouted)
N$115  (2 unrouted)
N$116  (2 unrouted)
N$117  (1 unrouted)
N$118  (1 unrouted)
N$119  (1 unrouted)
N$120  (1 unrouted)
N$121  (1 unrouted)
N$122  (1 unrouted)
N$123  (1 unrouted)
N$124  (2 unrouted)
N$125  (2 unrouted)
N$126  (2 unrouted)
N$127  (3 unrouted)
N$128  (1 unrouted)
N$129  (3 unrouted)
N$130  (2 unrouted)
N$131  (2 unrouted)
N$132  (4 unrouted)
N$133  (4 unrouted)
N$134  (1 unrouted)
N$135  (1 unrouted)
N$136  (1 unrouted)
N$137  (1 unrouted)
N$138  (1 unrouted)
N$139  (1 unrouted)
N$140  (1 unrouted)
N$141  (2 unrouted)
N$142  (2 unrouted)
N$143  (1 unrouted)
N$144  (1 unrouted)
N$145  (1 unrouted)
N$146  (1 unrouted)
N$147  (1 unrouted)
N$148  (1 unrouted)
N$149  (1 unrouted)
N$150  (1 unrouted)
N$151  (2 unrouted)
N$152  (2 unrouted)
N$153  (2 unrouted)
N$154  (2 unrouted)
N$155  (1 unrouted)
N$156  (1 unrouted)
N$157  (1 unrouted)
N$158  (1 unrouted)
N$159  (1 unrouted)
N$241  (2 unrouted)
N$242  (2 unrouted)
N$243  (2 unrouted)
N$244  (2 unrouted)
N$245  (1 unrouted)
N$246  (1 unrouted)
N$247  (1 unrouted)
N$248  (1 unrouted)
N$249  (1 unrouted)
N$250  (1 unrouted)
N$251  (1 unrouted)
N$252  (1 unrouted)
N$253  (1 unrouted)
N$254  (1 unrouted)
N$255  (1 unrouted)
N$256  (1 unrouted)
N$257  (1 unrouted)
N$258  (1 unrouted)
N$259  (1 unrouted)
N$260  (1 unrouted)
N$261  (1 unrouted)
N$262  (2 unrouted)
N$263  (1 unrouted)
N$268  (1 unrouted)
N$269  (1 unrouted)
N$270  (1 unrouted)
N$271  (1 unrouted)
N$272  (1 unrouted)
N$273  (2 unrouted)
N$274  (1 unrouted)
N$278  (2 unrouted)
N$279  (1 unrouted)
N$281  (3 unrouted)
N$282  (1 unrouted)
N$283  (2 unrouted)
N$284  (1 unrouted)
N$285  (1 unrouted)
N$286  (1 unrouted)
N$287  (1 unrouted)
N$289  (1 unrouted)
N$290  (1 unrouted)
N$291  (2 unrouted)
N$292  (1 unrouted)
N$293  (1 unrouted)
N$294  (2 unrouted)
N$295  (2 unrouted)
N$296  (1 unrouted)
N$297  (1 unrouted)
N$298  (1 unrouted)
N$299  (1 unrouted)
N$300  (1 unrouted)
N$301  (1 unrouted)
N$302  (1 unrouted)
N$303  (2 unrouted)
N$304  (2 unrouted)
N$305  (2 unrouted)
N$306  (2 unrouted)
N$307  (2 unrouted)
N$308  (1 unrouted)
N$309  (2 unrouted)
N$310  (1 unrouted)
N$311  (1 unrouted)
N$312  (1 unrouted)
N$313  (2 unrouted)
N$314  (2 unrouted)
N$315  (1 unrouted)
N$316  (1 unrouted)
N$317  (1 unrouted)
N$318  (2 unrouted)
N$319  (2 unrouted)
N$320  (2 unrouted)
N$321  (2 unrouted)
RFED  (2 unrouted)
RLOUT  (1 unrouted)
RMIX  (9 unrouted)
ROUT  (1 unrouted)
RROUT  (1 unrouted)
RST  (1 unrouted)
RT  (1 unrouted)
SC0  (1 unrouted)
SC1  (1 unrouted)
SCL  (1 unrouted)
SCLL  (1 unrouted)
SD0  (3 unrouted)
SD1  (3 unrouted)
SD2  (1 unrouted)
SD3  (1 unrouted)
SD4  (1 unrouted)
SD5  (1 unrouted)
SD6  (1 unrouted)
SD7  (1 unrouted)
SDA  (1 unrouted)
SDAA  (1 unrouted)
SFED  (3 unrouted)
V+  (via drill 0.5)  (9 unrouted)
  Top 0.406: v18.41,31.43 18.41,31.11 17.78,30.48 v13.65,30.48 | v13.02,28.57 v13.02,6.35 | v13.02,34.61 13.02,38.73 v13.34,39.05
  Bottom 0.406: 10.79,6.99 IC6.8 12.06,6.99 12.7,6.35 v13.02,6.35 | R16.2 R15.1 25.72,29.21 24.13,30.8 23.5,30.8 22.86,31.43 v18.41,31.43 18.41,31.75 17.78,32.38 17.78,38.73 15.88,40.64 14.92,40.64 | R29.2 R28.1 23.33,60.96 19.37,60.96 14.92,56.52 14.92,40.64 | v13.65,30.48 13.65,29.21 v13.02,28.57 | IC8.8 12.38,35.24 v13.02,34.61 | v13.34,39.05 14.92,40.64
V-  (via drill 0.5)  (25 unrouted)
  Top 0.406: v17.78,9.53 17.78,16.19 v16.83,17.14
  Bottom 0.406: IC6.4 17.14,3.17 17.78,3.81 v17.78,9.53 | v16.83,17.14 16.83,26.35 15.88,27.3 15.88,31.37 IC8.4
VCC  (20 unrouted)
